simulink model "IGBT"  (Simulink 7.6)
settings: Solver=ode23tb  StartTime=0.0  StopTime=50e-3  RelTol=1e-3
InitFcn:
  | clear all
  | close all
  | clc
  | 
  | delete *.mat
StopFcn:
  | close all
  | load IGBT_u.mat
  | plot(x(1,:),x(2,:),x(1,:),x(3,:))
  | grid
  | title('Tension entrée/sortie circuit à IGBT')
  | xlabel('temps')
  | 
  | close all
  | load IGBT_i.mat
  | plot(y(1,:),y(2,:))
  | grid
  | title('Courant sortie circuit à IGBT')
  | xlabel('temps')
  | 
  | delete *.mat
libraries: powerlib x10

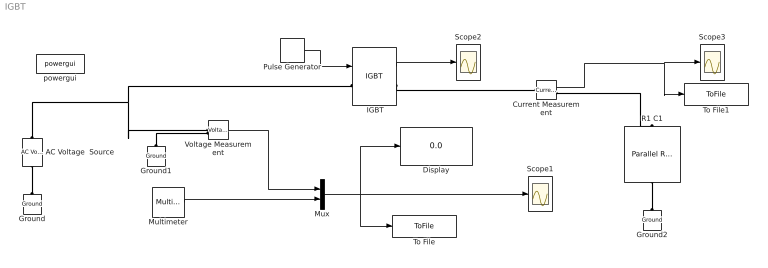
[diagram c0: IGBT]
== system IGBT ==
  " IGBT" : powerlib/Power Electronics/IGBT  DialogController=POWERSYS.PowerSysDialog  SystemSampleTime=-1  Ron=0.01  Lon=0  Vf=1  Tf=1e-6  Tt=1e-6  IC=0  Rs=10000  Cs=inf  Measurements=on
  AC Voltage  Source : powerlib/Electrical Sources/AC Voltage Source  DialogController=POWERSYS.PowerSysDialog  SystemSampleTime=-1  Amplitude=100  Phase=0  Frequency=60  SampleTime=0  Measurements=None
  Current Measurement : powerlib/Measurements/Current Measurement  DialogController=POWERSYS.PowerSysDialog  SystemSampleTime=-1  PhasorSimulation=off  OutputType=Complex  PSBequivalent=0
  Display : Display
  Ground : powerlib/Elements/Ground  DialogController=POWERSYS.PowerSysDialog  PhysicalDomain=powersysdomain  SubClassName=unknown  LeftPortType=p1  RightPortType=p1  LConnTagsString=a
  Ground1 : powerlib/Elements/Ground  DialogController=POWERSYS.PowerSysDialog  PhysicalDomain=powersysdomain  SubClassName=unknown  LeftPortType=p1  RightPortType=p1  LConnTagsString=a
  Ground2 : powerlib/Elements/Ground  DialogController=POWERSYS.PowerSysDialog  PhysicalDomain=powersysdomain  SubClassName=unknown  LeftPortType=p1  RightPortType=p1  LConnTagsString=a
  Multimeter : powerlib/Measurements/Multimeter  SystemSampleTime=-1  PhasorSimulation=off  OutputType=Complex  sel=1  L=2  Gain=1  yselected={'Ub: R1 C1'};  PSBOutputType=1  PSBequivalent=0  AxesSetting=[0,0.1,-100,100]  Display=0  SavedBlockNames=-11
  Mux : Mux  Inputs=2
  Pulse Generator : DiscretePulseGenerator  PulseType=Time based  Period=1/60  PulseWidth=50
  R1 C1 : powerlib/Elements/Parallel RLC Branch  DialogController=POWERSYS.PowerSysDialog  PhysicalDomain=powersysdomain  SubClassName=unknown  LeftPortType=p1  RightPortType=p1  LConnTagsString=a  RConnTagsString=__new0  BranchType=RC  Resistance=50  Inductance=1.0  SetiL0=off  InitialCurrent=0  Capacitance=25e-06  Setx0=off  InitialVoltage=0  Measurements=Branch voltage and current
  Scope1 : Scope
  Scope2 : Scope
  Scope3 : Scope
  To File : ToFile  Filename=IGBT_u  MatrixName=x
  To File1 : ToFile  Filename=IGBT_i  MatrixName=y
  Voltage Measurement : powerlib/Measurements/Voltage Measurement  DialogController=POWERSYS.PowerSysDialog  SystemSampleTime=-1  PhasorSimulation=off  OutputType=Complex  PSBequivalent=0
  powergui : powerlib/powergui  SystemSampleTime=-1  SimulationMode=Continuous  SampleTime=0  frequency=60  SPID=off  DisableSnubberDevices=off  DisableRonSwitches=off  DisableVfSwitches=off  SwTol=0  Interpol=off  frequencyindice=0  echomessages=off  HookPort=off  DisplayEquations=off  FunctionMessages=off  EnableUseOfTLC=off  x0status=blocks  RestoreLinks=warning  ResistiveCurrentMeasurement=off  Frange=[0:2:500]  Ylog=off  Xlog=on  ShowGrid=off  save=off  variable=ZData  ZoomFFT=on  StartTime=0.0  cycles=1  DisplayStyle=1  fundamental=60  FreqAxis=off  MaxFrequency=1000  frequencyindicesteady=1  RmsSteady=1  display=off  Ts=0  methode=off
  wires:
  Multimeter/1 -> Mux/2
  Mux/1 -> Scope1/1, Display/1, To File/1
  Voltage Measurement/1 -> Mux/1
  Pulse Generator/1 -> " IGBT"/1
  " IGBT"/1 -> Scope2/1
  Current Measurement/1 -> Scope3/1, To File1/1
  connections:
  AC Voltage  Source/LConn1 -- Ground/LConn1
  R1 C1/RConn1 -- Ground2/LConn1
  AC Voltage  Source/RConn1 -- " IGBT"/LConn1 -- Voltage Measurement/LConn1
  Ground1/LConn1 -- Voltage Measurement/LConn2
  " IGBT"/RConn1 -- Current Measurement/LConn1
  Current Measurement/RConn1 -- R1 C1/LConn1
